FUNCTION_BLOCK FB_SBOwControl EXTENDS FB_AsyncServiceResultClass
VAR
	_ipClient 	: I_ScsmClientClass;	
	_ipCtrl 	: I_AcsiCommonControllableDataClass;(* interface pointer to controllable data object *)

	_ctlVal		: U_AcsiCtlVal;
	_operTm 	: T_UtcTime;
	_origin		: ST_AcsiOriginator := ( orCat := E_AcsiOrCategory.StationControl, orIdent := [16#BE,16#CF,16#61,16#85] );
	_ctlNum		: USINT;
	_bTest 		: BOOL;
	_eCheck		: E_AcsiCheck;
	_eControl	: E_AcsiCtlService;
	
	_nInvokeID 	: UDINT;
	_ipResult 	: I_AsyncServiceResultClass;

	_tmpCtlVal	: U_AcsiCtlVal;
	_bMxVal		: BOOL;
	state 		: UDINT;
END_VAR

METHOD APC : BOOL
VAR_INPUT
	ipClient 	: I_ScsmClientClass;	
	ipCtrl 		: I_AcsiCommonControllableDataClass;
	ctlVal		: REAL;
	eControl	: E_AcsiCtlService;
END_VAR
VAR_OUTPUT
	ipResult 	: I_AsyncServiceResultClass;
END_VAR
_tmpCtlVal.APC.f:= ctlVal;
APC:= Request(ipClient:=ipClient, ipCtrl:=ipCtrl, ctlVal:=_tmpCtlVal, eControl:=eControl, bMxVal:=TRUE, ipResult=>ipResult);
END_METHOD

METHOD BAC : BOOL
VAR_INPUT
	ipClient 	: I_ScsmClientClass;	
	ipCtrl 		: I_AcsiCommonControllableDataClass;
	ctlVal		: E_AcsiTcmd;
	eControl 	: E_AcsiCtlService;
END_VAR
VAR_OUTPUT
	ipResult 	: I_AsyncServiceResultClass;
END_VAR
_tmpCtlVal.BAC:= ctlVal;
BAC:= Request(ipClient:=ipClient, ipCtrl:=ipCtrl, ctlVal:=_tmpCtlVal, eControl:=eControl, bMxVal:=TRUE, ipResult=>ipResult);
END_METHOD

METHOD BSC : BOOL
VAR_INPUT
	ipClient 	: I_ScsmClientClass;	
	ipCtrl 		: I_AcsiCommonControllableDataClass;
	ctlVal		: E_AcsiTcmd;
	eControl 	: E_AcsiCtlService;
END_VAR
VAR_OUTPUT
	ipResult 	: I_AsyncServiceResultClass;
END_VAR
_tmpCtlVal.BSC:= ctlVal;
BSC:= Request(ipClient:=ipClient, ipCtrl:=ipCtrl, ctlVal:=_tmpCtlVal, eControl:=eControl, bMxVal:=FALSE, ipResult=>ipResult);
END_METHOD

PROPERTY bTest : BOOL
SET
_bTest:= bTest;
END_SET
END_PROPERTY

METHOD Clear
VAR_INPUT
	ipReason : I_ServiceErrorClass;
END_VAR
IF SUPER^.IsBusy() THEN
	SUPER^.SetAborted(ipReason:=ipReason);
END_IF
state:= 0;
END_METHOD

PROPERTY ctlNum : USINT
GET
ctlNum:= _ctlNum;
END_GET
END_PROPERTY

METHOD DPC : BOOL
VAR_INPUT
	ipClient 	: I_ScsmClientClass;	
	ipCtrl 		: I_AcsiCommonControllableDataClass;
	ctlVal		: BOOL;
	eControl 	: E_AcsiCtlService;
END_VAR
VAR_OUTPUT
	ipResult 	: I_AsyncServiceResultClass;
END_VAR
_tmpCtlVal.DPC:= ctlVal;
DPC:= Request(ipClient:=ipClient, ipCtrl:=ipCtrl, ctlVal:=_tmpCtlVal, eControl:=eControl, bMxVal:=FALSE, ipResult=>ipResult);
END_METHOD

PROPERTY eCheck : E_AcsiCheck
SET
_eCheck:= eCheck;
END_SET
END_PROPERTY

METHOD ENC_Mod : BOOL
VAR_INPUT
	ipClient 	: I_ScsmClientClass;	
	ipCtrl 		: I_AcsiCommonControllableDataClass;
	ctlVal		: E_AcsiMod;
	eControl : E_AcsiCtlService;
END_VAR
VAR_OUTPUT
	ipResult 	: I_AsyncServiceResultClass;
END_VAR
_tmpCtlVal.ENC.Mode:= ctlVal;
ENC_Mod:= Request(ipClient:=ipClient, ipCtrl:=ipCtrl, ctlVal:=_tmpCtlVal, eControl:=eControl, bMxVal:=FALSE, ipResult=>ipResult);
END_METHOD

METHOD Execute : BOOL
CASE state OF
	0:RETURN;(* idle state *)

	(*--------------------- Verify status (optional) -----------------------------------*)
	1: (* Read control status information e.g.: "IEDLD1/CSWI1.ST.Pos" (stVal, q, t, stSeld, ...)*)
		state:= SEL(_ipClient.GetDataValuesReq(ipData:=_ipCtrl, eFC:=SEL(_bMxVal, E_AcsiFc.ST_, E_AcsiFc.MX), hUser:=0, ipSink:=0, nInvokeID=>_nInvokeID, ipResult=>_ipResult), 100, 2); 
	2:
		IF _ipResult <> 0 THEN
			_ipResult.Execute();
			IF NOT _ipResult.IsBusy() THEN
				state:= SEL(_ipResult.IsCompleted(), 100, 10);
			END_IF
		END_IF
		
	(*--------------------- Verify config (optional) ------------------------------------*)
	10: (* Read control configuration e.g.: "IEDLD1/CSWI1.CF.Pos" (ctlModel, sboTimeout, pulseConfig, ...)*)
		state:= SEL(_ipClient.GetDataValuesReq(ipData:=_ipCtrl, eFC:=E_AcsiFc.CF, hUser:=0, ipSink:=0, nInvokeID=>_nInvokeID, ipResult=>_ipResult), 100, 11); 
	11:
		IF _ipResult <> 0 THEN
			_ipResult.Execute(); 
			IF NOT _ipResult.IsBusy() THEN
				state:= SEL(_ipResult.IsCompleted(), 100, 12);
			END_IF
		END_IF

	12: (* Check ctlModel, stSeld (optional) *)
		IF (_ipCtrl <> 0) AND_THEN (_ipCtrl.ipSBOw <> 0) AND_THEN (_ipCtrl.ipCtlModel <> 0) AND_THEN (_ipCtrl.ipCtlModel.eValue = E_AcsiCtlModels.SBOWithEnhancedSecurity) THEN
			IF (_eControl = E_AcsiCtlService.Select) OR (_eControl = E_AcsiCtlService.SelectAndOperate) THEN 
				IF (_ipCtrl.ipStSeld <> 0) AND_THEN _ipCtrl.ipStSeld.bValue THEN
					IF _eControl = E_AcsiCtlService.Select THEN
						_eControl:= E_AcsiCtlService.None;
						state:= 50;(* update status *)
					ELSIF _eControl = E_AcsiCtlService.SelectAndOperate THEN
						_eControl:= E_AcsiCtlService.Operate;
						state:= 30;(* operate, update status  *)
					END_IF
				ELSE
					state:= 20;(* select | select&operate, update status *)				
				END_IF
			ELSIF _eControl = E_AcsiCtlService.Operate THEN 
				state:= 30;(* operate, update status *)
			ELSIF _eControl = E_AcsiCtlService.Cancel THEN
				state:= 40;(* cancel, update status *) 
			END_IF	
		ELSE(* fatal error *)
			state:= 90;
		END_IF
		
	(*--------------------- Select with value (SBOw) ----------------------------------------------------*)
	20: (* Write "SBOw" structure e.g.: "IEDLD1/CSWI1.CO.SBOw" (ctlVal, operTm, origin, ctlNum, T, Test, Check) *)
		IF (_eControl = E_AcsiCtlService.Select) OR (_eControl = E_AcsiCtlService.SelectAndOperate) THEN
			_ctlNum:= _ctlNum + 1; 
			state:= SEL(_ipClient.ControlSelectWithValueReq(ipCtrl:=_ipCtrl, ctlVal:=_ctlVal, operTm:=_operTm, origin:=_origin, ctlNum:=_ctlNum, bTest:=_bTest, eCheck:=_eCheck, hUser:=0, ipSink:=0, nInvokeID=>_nInvokeID, ipResult=>_ipResult), 100, 21);
		ELSE(* operate  *)
			state:= 30;			
		END_IF
	21:
		IF _ipResult <> 0 THEN
			_ipResult.Execute();
			IF NOT _ipResult.IsBusy() THEN
				state:= SEL( _ipResult.IsCompleted(), 100, 30);
			END_IF
		END_IF
		
	(*--------------------- Operate ----------------------------------------------------*)
	30: (* Write "Oper" structure e.g.: "IEDLD1/CSWI1.CO.Pos.Oper" (ctlVal, operTm, origin, ctlNum, T, Test, Check) *)
		IF (_eControl = E_AcsiCtlService.Operate) OR (_eControl = E_AcsiCtlService.SelectAndOperate) THEN
			state:= SEL(_ipClient.ControlOperateReq(ipCtrl:=_ipCtrl, ctlVal:=_ctlVal, operTm:=_operTm, origin:=_origin, ctlNum:=_ctlNum, bTest:=_bTest, eCheck:=_eCheck, hUser:=0, ipSink:=0, nInvokeID=>_nInvokeID, ipResult=>_ipResult), 100, 31);
		ELSE
			state:= 40;
		END_IF			
	31:
		IF _ipResult <> 0 THEN
			_ipResult.Execute();
			IF NOT _ipResult.IsBusy() THEN
				state:= SEL(_ipResult.IsCompleted(), 100, 40);
			END_IF
		END_IF

	(*--------------------- Cancel ----------------------------------------------------*)
	40: (* Write "Cancel" structure e.g.: "IEDLD1/CSWI1.CO.Pos.Cancel" (ctlVal, operTm, origin, ctlNum, T, Test )*)
		IF (_eControl = E_AcsiCtlService.Cancel) THEN
			state:= SEL(_ipClient.ControlCancelReq(ipCtrl:=_ipCtrl, ctlVal:=_ctlVal, operTm:=_operTm, origin:=_origin, ctlNum:=_ctlNum, bTest:=_bTest, hUser:=0, ipSink:=0, nInvokeID=>_nInvokeID, ipResult=>_ipResult), 100, 41);
		ELSE
			state:= 50;
		END_IF			
	41:
		IF _ipResult <> 0 THEN
			_ipResult.Execute();
			IF NOT _ipResult.IsBusy() THEN
				state:= SEL(_ipResult.IsCompleted(), 100, 50);
			END_IF
		END_IF
		
		
	(*--------------------- Update status (optional) -----------------------------------*)
	50: (* Read control status information e.g.: "IEDLD1/CSWI1.ST.Pos" (stVal, q, t, ...) *)		
		state:= SEL(_ipClient.GetDataValuesReq(ipData:=_ipCtrl, eFC:=SEL(_bMxVal, E_AcsiFc.ST_, E_AcsiFc.MX), hUser:=0, ipSink:=0, nInvokeID=>_nInvokeID, ipResult=>_ipResult), 100, 51); 
	51:
		IF _ipResult <> 0 THEN
			_ipResult.Execute();
			IF NOT _ipResult.IsBusy() THEN
				state:= SEL(_ipResult.IsCompleted(), 100, 80);
			END_IF
		END_IF
	
	80: (* Completed *)
		state:= 0;
		SUPER^.SetCompleted();

	90: (* Fatal error *)
		state:= 0;
		SUPER^.SetFailedEx(stError:=TC_EVENTS.TcAcsiEventClass.AccessViolation);

	100: (* Failed or aborted *)
		state:= 0;
		SUPER^.CopyFrom(ipSource:=_ipResult);
END_CASE
Execute:= TRUE;
END_METHOD

METHOD INC : BOOL
VAR_INPUT
	ipClient 	: I_ScsmClientClass;	
	ipCtrl 		: I_AcsiCommonControllableDataClass;
	ctlVal		: DINT;
	eControl	: E_AcsiCtlService;
END_VAR
VAR_OUTPUT
	ipResult 	: I_AsyncServiceResultClass;
END_VAR
_tmpCtlVal.INC:= ctlVal;
INC:= Request(ipClient:=ipClient, ipCtrl:=ipCtrl, ctlVal:=_tmpCtlVal, eControl:=eControl, bMxVal:=FALSE, ipResult=>ipResult);
END_METHOD

METHOD ISC : BOOL
VAR_INPUT
	ipClient 	: I_ScsmClientClass;	
	ipCtrl 		: I_AcsiCommonControllableDataClass;
	ctlVal		: SINT(-64..63);
	eControl	: E_AcsiCtlService;
END_VAR
VAR_OUTPUT
	ipResult 	: I_AsyncServiceResultClass;
END_VAR
_tmpCtlVal.ISC:= ctlVal;
ISC:= Request(ipClient:=ipClient, ipCtrl:=ipCtrl, ctlVal:=_tmpCtlVal, eControl:=eControl, bMxVal:=FALSE, ipResult=>ipResult);
END_METHOD

METHOD OnCommandTerminationInd
VAR_INPUT
	ipCtrl	: I_AcsiCommonControllableDataClass;
END_VAR
END_METHOD

METHOD OnControlCnf
VAR_INPUT
	ipCtrl	: I_AcsiCommonControllableDataClass;
END_VAR
END_METHOD

METHOD OnLastApplErrorInd
VAR_INPUT
	ipCtrl	: I_AcsiCommonControllableDataClass;
END_VAR
END_METHOD

PROPERTY operTm : T_UtcTime
SET
_operTm:= operTm;
END_SET
END_PROPERTY

PROPERTY origin : ST_AcsiOriginator
SET
_origin:= origin;
END_SET
END_PROPERTY

METHOD PRIVATE Request : BOOL
VAR_INPUT
	ipClient 	: I_ScsmClientClass;	
	ipCtrl 		: I_AcsiCommonControllableDataClass;
	ctlVal		: U_AcsiCtlVal;
	eControl	: E_AcsiCtlService;
	bMxVal		: BOOL;(* TRUE => status information is analogue value "mxVal", FALSE => status information is not analogue value "stVal" *)
END_VAR
VAR_OUTPUT
	ipResult : I_AsyncServiceResultClass := THIS^;
END_VAR
IF Request:= SUPER^.IsBusy() THEN
	RETURN;
END_IF

IF (ipClient = 0) OR (ipCtrl = 0) OR_ELSE (ipCtrl.ipOper = 0) OR_ELSE (ipCtrl.ipSBOw = 0) OR_ELSE (ipCtrl.ipCancel = 0) OR_ELSE (ipCtrl.ipCtlModel = 0) THEN
	SUPER^.SetFailedEx(stError:=TC_EVENTS.TcAcsiEventClass.AccessViolation);
	RETURN;
END_IF 

IF eControl = E_AcsiCtlService.None THEN
	SUPER^.SetCompleted();
	RETURN;
END_IF

_ipClient:= ipClient;
_ipCtrl:= ipCtrl;
_ctlVal:= ctlVal;
_eControl:= eControl;
_bMxVal:= bMxVal;

SUPER^.SetBusy();
state:= 1;
Request:= TRUE;
END_METHOD

METHOD SPC : BOOL
VAR_INPUT
	ipClient 	: I_ScsmClientClass;	
	ipCtrl 		: I_AcsiCommonControllableDataClass;
	ctlVal		: BOOL;
	eControl	: E_AcsiCtlService;
END_VAR
VAR_OUTPUT
	ipResult 	: I_AsyncServiceResultClass;
END_VAR
_tmpCtlVal.SPC:= ctlVal;
SPC:= Request(ipClient:=ipClient, ipCtrl:=ipCtrl, ctlVal:=_tmpCtlVal, eControl:=eControl, bMxVal:=FALSE, ipResult=>ipResult);
END_METHOD

END_FUNCTION_BLOCK
